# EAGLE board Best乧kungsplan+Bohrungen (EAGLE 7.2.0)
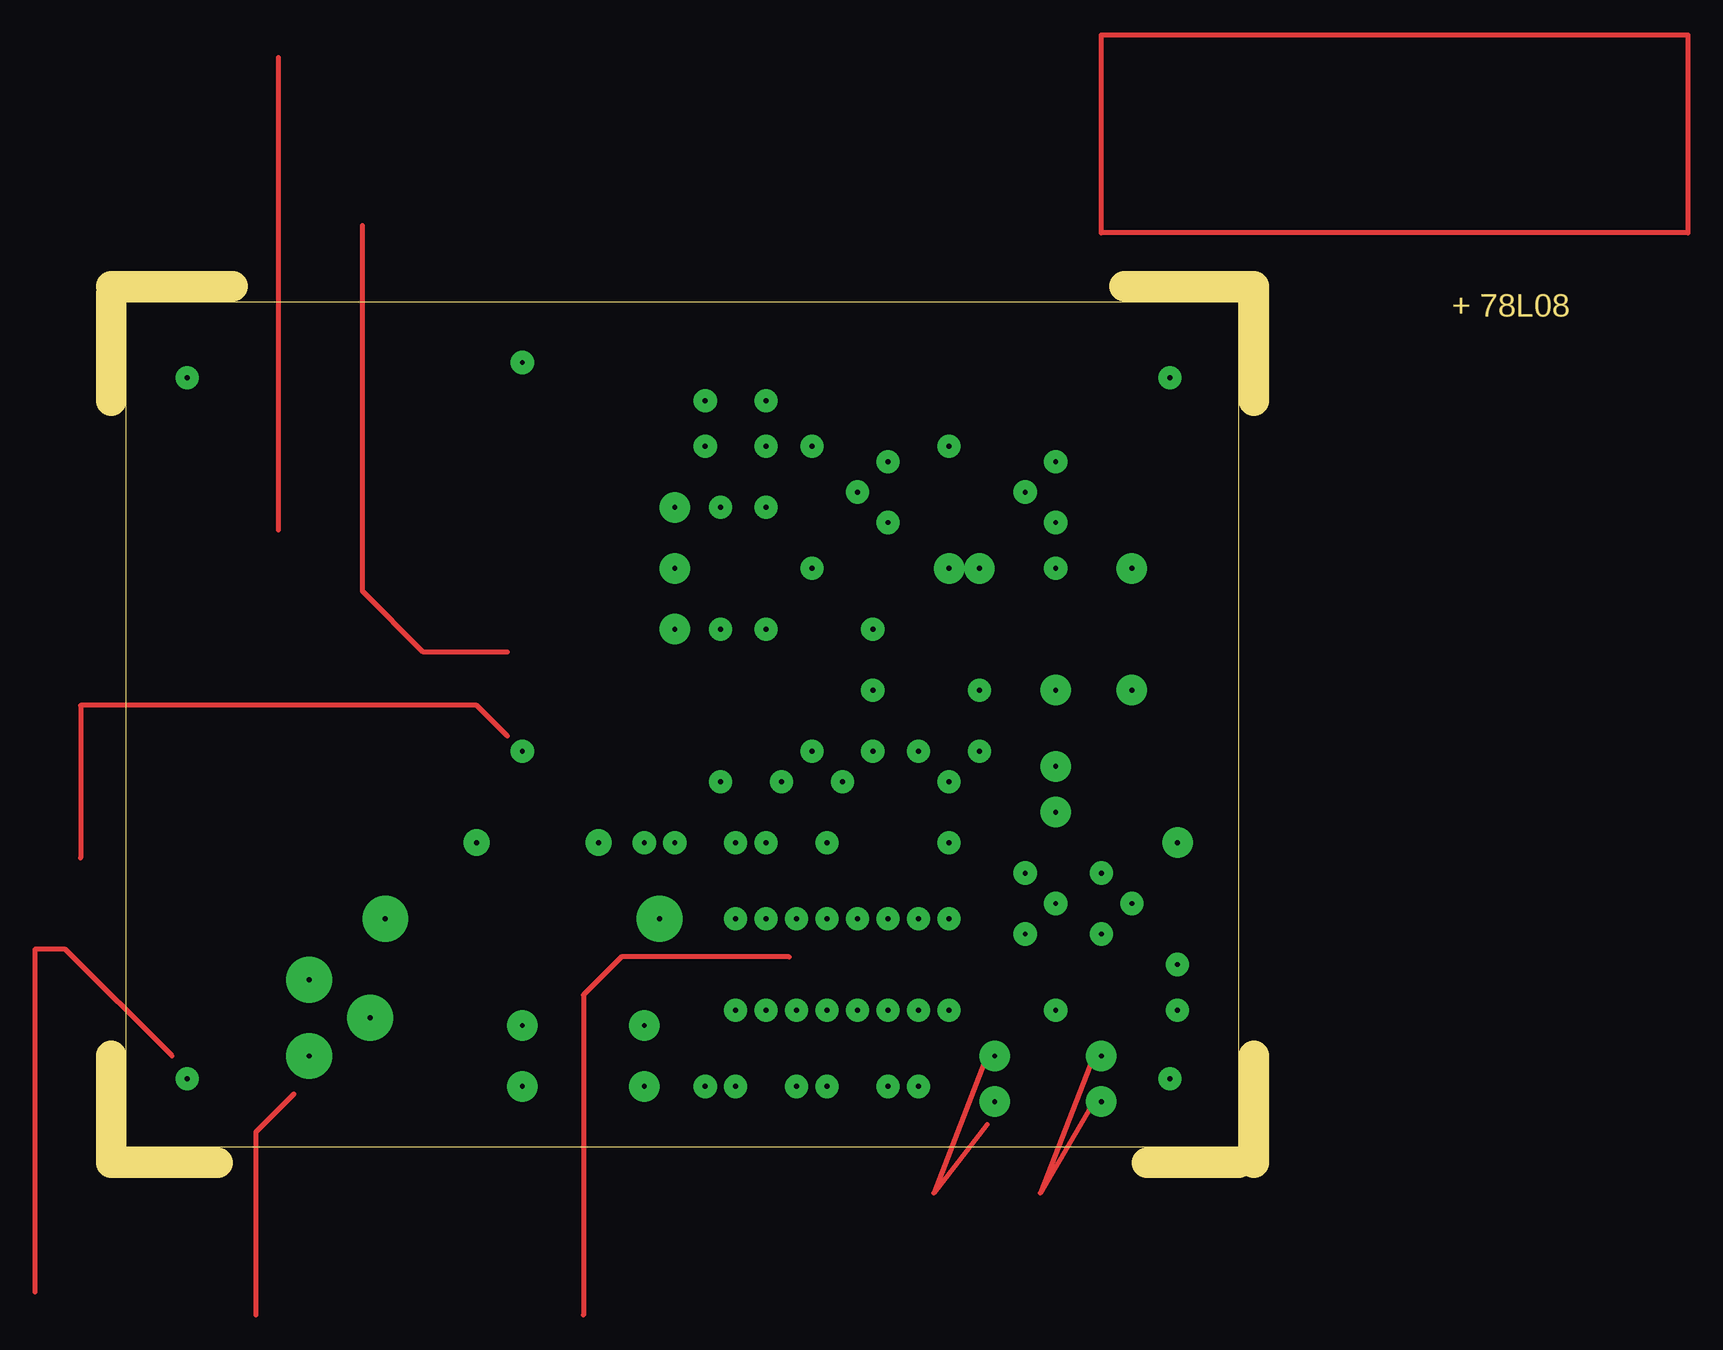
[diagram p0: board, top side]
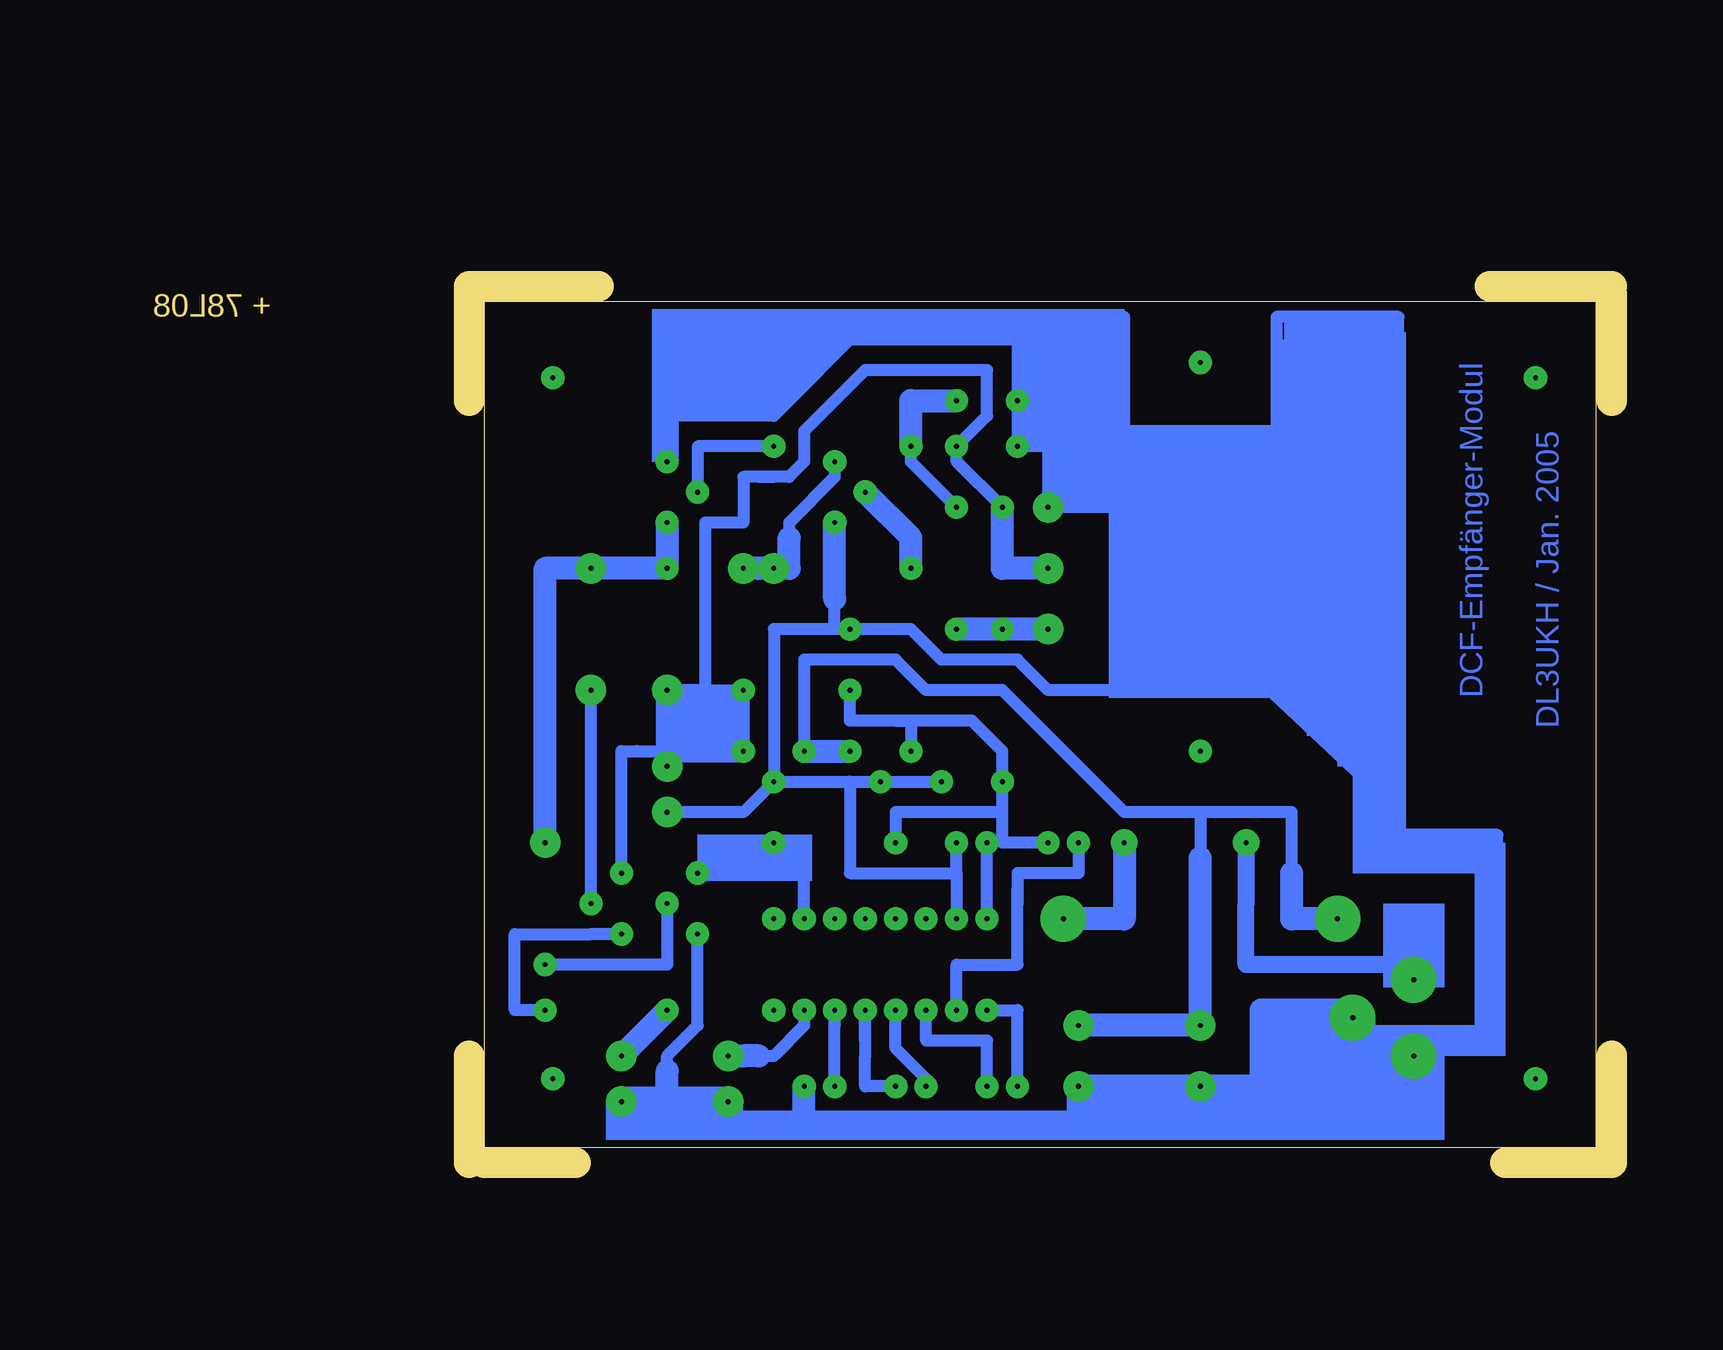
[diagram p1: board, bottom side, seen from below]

Size 95.25 x 73.02 mm. Coordinates in mm from the lower left corner, seen from the top.
Outline: 0,8.89 0,0 8.89,0
Outline: 0,72.39 0,63.5
Outline: 93.98,0 86.36,0
Outline: 95.25,0 95.25,8.89
Outline: 95.25,72.39 95.25,63.5
Outline: 0,73.02 10.16,73.02
Outline: 95.25,72.71 95.25,73.02 84.45,73.02
Outline: 1.27,71.75 93.98,71.75 93.98,1.27 1.27,1.27 1.27,71.75
Copper layers (1*16): Top 0.035mm / dielectric 1.5mm / Bottom 0.035mm
Design rules "default": minimum track width 10mil, minimum drill 24mil, track to track 8mil, track to pad 8mil, pad to pad 8mil, via to via 8mil, smd to smd 8mil, copper to edge 40mil, drill to drill 8mil, minimum pad ring 10mil, minimum via ring 8mil, stop-mask expansion 4mil, vias tented up to drill 0mil, thermal gap 10mil

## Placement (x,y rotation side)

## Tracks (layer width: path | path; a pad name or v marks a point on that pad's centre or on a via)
S$1  (via drill 0.41 pad 1.93)
  other vias: 6.35,6.98
S$2  (via drill 0.41 pad 1.93)
  other vias: 88.27,6.98
S$3  (via drill 0.41 pad 1.93)
  other vias: 88.27,65.41
S$4  (via drill 0.41 pad 1.93)
  other vias: 6.35,65.41
S$5
  Top 0.406: 33.02,42.55 26.04,42.55 20.95,47.62 20.95,78.1
S$6  (via drill 0.41 pad 2.18)
  Bottom 1.422: 16.51,16.51 30.48,16.51 30.48,21.59 v30.48,26.67
S$7  (via drill 0.41 pad 1.93)
  other vias: 34.29,34.29
S$8  (via drill 0.41 pad 1.93)
  other vias: 34.29,66.67
S$9  (via drill 0.41 pad 3.81)
  Bottom 1.93: v16.51,15.24 17.78,16.51
S$10
  Bottom 1.016: 11.43,10.79 14.61,10.79
S$11  (via drill 0.41 pad 3.81)
  other vias: 21.59,12.06
S$12  (via drill 0.41 pad 1.93)
  Bottom 1.016: v44.45,26.67 44.45,24.13 49.53,24.13 49.53,21.59 | 49.53,21.59 49.53,22.86 | v54.61,12.7 54.61,16.51 49.53,16.51 49.53,21.59
S$13  (via drill 0.41 pad 2.18, 0.41 pad 3.81)
  Bottom 1.93: v40.64,26.67 40.64,20.32 v45.72,20.32
S$14  (via drill 0.41 pad 1.93, 0.41 pad 2.54, 0.41 pad 3.81)
  Bottom 1.016: v63.5,34.29 v67.31,34.29 67.31,41.91 59.69,41.91 57.15,39.37 50.8,39.37 40.64,29.21 38.1,29.21 | 34.29,29.21 34.29,25.4 | 38.1,29.21 39.37,29.21 | 34.29,29.21 26.67,29.21 26.67,24.13 | 34.29,29.21 38.1,29.21
  Bottom 1.93: v44.45,11.43 v34.29,11.43 34.29,25.4 | v22.86,20.32 26.67,20.32 26.67,24.13 | v67.31,34.29 v63.5,34.29
S$15
  Bottom 1.93: 19.05,31.11 29.21,40.64
S$16  (via drill 0.41 pad 1.93, 0.41 pad 2.54)
  Bottom 1.016: v46.99,44.45 v50.8,44.45 v54.61,44.45
  Bottom 1.93: v46.99,44.45 v54.61,44.45
S$17  (via drill 0.41 pad 1.93)
  Bottom 1.93: v62.23,55.88 58.42,52.07 v58.42,49.53
S$18  (via drill 0.41 pad 1.93)
  Bottom 1.016: v52.07,6.35 52.07,10.16 57.15,10.16 v57.15,12.7
S$19  (via drill 0.41 pad 1.93)
  other vias: 76.2,19.05
S$20  (via drill 0.41 pad 1.93)
  Bottom 1.016: 64.77,11.43 v64.77,12.7 v64.77,6.35
S$21  (via drill 0.41 pad 1.93)
  Bottom 1.016: v54.61,54.61 58.42,58.42 v58.42,59.69
  Bottom 1.93: v54.61,63.5 58.42,63.5 v58.42,59.69
S$22  (via drill 0.41 pad 1.93, 0.41 pad 2.54, 0.41 pad 3.81)
  Bottom 1.016: 76.2,19.05 76.2,11.43 78.74,8.89 78.74,7.62 | 78.74,3.81 78.74,5.08 | 78.74,3.81 73.66,3.81 67.31,3.81 44.45,3.81 | 78.74,3.81 82.55,3.81 v82.55,5.08
  Bottom 1.93: 78.74,5.08 78.74,7.62 | 67.31,3.81 v67.31,6.35 | 44.45,5.08 v44.45,6.35 v34.29,6.35 | v82.55,5.08 v73.66,5.08 | 44.45,5.08 44.45,3.81 34.29,3.81 | 34.29,5.08 44.45,5.08 | 34.29,5.08 34.29,3.81 | 34.29,3.81 16.51,3.81 16.51,5.08 | 34.29,5.08 v34.29,6.35 | 16.51,6.35 29.21,6.35 | 29.21,6.35 v34.29,6.35 | 16.51,6.35 v16.51,8.89 | 16.51,5.08 21.59,5.08 | 21.59,5.08 34.29,5.08 | 16.51,5.08 16.51,6.35 | 21.59,5.08 21.59,7.62 | 21.59,12.06 21.59,12.7 29.21,12.7 29.21,6.35
  Bottom 2.54: 73.66,3.81 v73.66,5.08 v82.55,5.08 | 21.59,8.89 21.59,7.62
  Bottom 3.81: 21.59,12.06 21.59,8.89
S$23  (via drill 0.41 pad 1.93)
  other vias: 69.85,12.7
S$24  (via drill 0.41 pad 1.93)
  Bottom 1.016: v88.9,12.7 91.44,12.7 91.44,19.05 85.09,19.05 v82.55,19.05
S$25  (via drill 0.41 pad 1.93, 0.41 pad 2.54)
  Bottom 1.016: v85.09,21.59 v85.09,39.37
S$26  (via drill 0.41 pad 1.93)
  other vias: 57.15,20.32
S$27  (via drill 0.41 pad 1.93)
  other vias: 59.69,20.32
S$28  (via drill 0.41 pad 1.93)
  other vias: 62.23,20.32
S$29  (via drill 0.41 pad 1.93)
  other vias: 64.77,20.32
S$30  (via drill 0.41 pad 1.93)
  Bottom 1.016: v69.85,26.67 67.31,26.67 67.31,24.13 | v67.31,20.32 67.31,24.13 | 67.31,24.13 v76.2,24.13
S$31  (via drill 0.41 pad 1.93)
  other vias: 69.85,20.32
S$32  (via drill 0.41 pad 1.93)
  Bottom 1.016: v63.5,39.37 63.5,36.83 59.69,36.83 | v58.42,34.29 58.42,36.83 59.69,36.83 | 59.69,36.83 53.34,36.83 50.8,34.29 v50.8,31.75 50.8,29.21 | 50.8,29.21 50.8,26.67 v46.99,26.67 | 50.8,29.21 59.69,29.21 v59.69,26.67
S$33  (via drill 0.41 pad 1.93)
  Bottom 1.016: v52.07,20.32 v52.07,26.67
S$34
  Bottom 1.93: 66.67,69.21 71.12,64.77
S$35  (via drill 0.41 pad 1.93)
  Bottom 1.016: v59.69,12.7 59.69,9.53 57.15,6.98 v57.15,6.35
S$36  (via drill 0.41 pad 1.93)
  Bottom 1.016: v59.69,6.35 62.23,6.35 62.23,8.89 v62.23,12.7 62.23,10.16
S$37  (via drill 0.41 pad 1.93)
  Bottom 1.016: v49.53,6.35 49.53,12.7 v52.07,12.7
S$38  (via drill 0.41 pad 1.93)
  Bottom 1.016: v69.85,59.69 76.2,59.69 v76.2,55.88
S$39  (via drill 0.41 pad 1.93, 0.41 pad 2.54)
  Bottom 1.93: v88.9,26.67 88.9,49.53 v85.09,49.53 v78.74,49.53 v78.74,53.34
S$40  (via drill 0.41 pad 1.93, 0.41 pad 2.54)
  Bottom 1.016: v64.77,58.42 64.77,57.15 68.58,53.34 68.58,52.07 | 71.12,49.53 v72.39,49.53
  Bottom 1.93: v69.85,49.53 68.58,49.53 68.58,52.07 | v69.85,49.53 71.12,49.53 | v69.85,49.53 v72.39,49.53
S$41
  Bottom 1.93: 27.94,40.64 24.13,36.83
S$42  (via drill 0.41 pad 1.93)
  Bottom 1.016: v78.74,21.59 78.74,16.51 v88.9,16.51
S$43  (via drill 0.41 pad 1.93, 0.41 pad 2.54)
  Bottom 1.016: v67.31,12.7 67.31,11.43 69.85,8.89 71.12,8.89
  Bottom 1.93: 71.12,8.89 72.39,8.89 v73.66,8.89
S$44  (via drill 0.41 pad 1.93, 0.41 pad 2.54)
  Bottom 1.93: v78.74,12.7 v82.55,8.89
S$45  (via drill 0.41 pad 1.93, 0.41 pad 2.54)
  Bottom 1.016: 54.61,24.13 v54.61,26.67 | 54.61,24.13 v54.61,20.32 | 54.61,24.13 63.5,24.13 63.5,31.75 | v55.88,31.75 v60.96,31.75 63.5,31.75 | v78.74,29.21 72.39,29.21 v69.85,31.75 | v69.85,31.75 63.5,31.75 | v69.85,31.75 69.85,44.45 64.77,44.45 | 64.77,44.45 64.77,46.99 | 64.77,44.45 v63.5,44.45 58.42,44.45 55.88,41.91 49.53,41.91 46.99,39.37 40.64,39.37 40.64,40.64 | 78.74,63.5 73.66,68.58 69.85,68.58 | v49.53,63.5 v49.53,59.69 46.99,59.69 | 69.85,68.58 69.85,62.23 | 49.53,68.58 64.77,68.58 69.85,68.58 | 49.53,68.58 v49.53,63.5 | 46.99,63.5 v49.53,63.5 | 46.99,59.69 v46.99,54.61 40.64,54.61 | 46.99,59.69 46.99,63.5 | 40.64,54.61 39.37,54.61 | 40.64,54.61 46.99,59.69 | 46.99,68.58 46.99,63.5 | 46.99,68.58 49.53,68.58 | 46.99,68.58 40.64,68.58 40.64,60.96 | 40.64,60.96 40.64,57.15 40.64,70.48 78.74,70.48 | 40.64,60.96 27.94,60.96 27.94,70.48 17.78,70.48 17.78,27.3 9.53,27.3 9.53,12.7 | 69.85,62.23 62.23,69.85 | 69.85,62.23 78.74,62.23
  Bottom 1.93: 64.77,46.99 v64.77,53.34 | 78.74,63.5 78.74,62.23 v78.74,58.42 | 40.64,40.64 40.64,54.61 40.64,57.15 | 64.77,68.58 70.48,62.87
S$46
  Top 0.406: 56.52,17.14 42.55,17.14 39.37,13.97 39.37,-12.7
S$47  (via drill 0.41 pad 1.93, 0.41 pad 2.54)
  Bottom 1.016: 82.55,34.29 81.28,34.29 | v82.55,24.13 82.55,34.29 | v72.39,34.29 v72.39,39.37 75.56,39.37 | 75.56,39.37 v78.74,39.37 | 75.56,39.37 75.56,53.34 72.39,53.34 72.39,57.15 71.12,57.15 | 71.12,57.15 69.85,57.15 | 71.12,57.15 68.58,57.15 67.31,58.42 67.31,60.96 62.23,66.04 52.07,66.04 52.07,62.23 v54.61,59.69 54.61,58.42 v50.8,54.61 | 82.55,34.29 78.74,34.29
  Bottom 1.93: 78.74,34.29 v78.74,33.02 | v72.39,34.29 78.74,34.29 | v78.74,39.37 78.74,34.29 | v50.8,54.61 50.8,49.53 v46.99,49.53
S$48
  Bottom 1.016: 41.28,69.21 78.74,69.21
S$49
  Top 0.406: 73.02,8.89 68.58,-2.54 73.02,3.17
S$50
  Top 0.406: 81.91,8.89 77.47,-2.54 81.91,5.08
S$51
  Top 0.406: 33.02,35.56 30.48,38.1 -2.54,38.1 -2.54,25.4
S$52
  Top 0.406: 5.08,8.89 -3.81,17.78 -6.35,17.78 -6.35,-10.79
S$53
  Top 0.406: 13.97,52.71 13.97,92.08
S$54
  Top 0.406: 15.24,5.71 12.06,2.54 12.06,-12.7
S$55
  Top 0.406: 82.55,93.98 131.45,93.98 131.45,77.47 82.55,77.47 82.55,93.98
(copper drawn outside any net)
  shapes: Bottom area x42

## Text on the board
Bottom: DCF-Empfänger-Modul | DL3UKH / Jan. 2005
Pads: AUF BESTÜCKUNGS-SEITE GESEHEN
Dimension: + 78L08
tOrigins: Es ist keine Leiterplatten-Brücke notwendig ! | Freien Platz NICHT für Ferrit-Ant. | BOHRUNGEN | nutzen. Ant. außerhalb platzieren !!! | Alles mit 0,8mm bohren. | Anschluß-Drähte verlängern | alle Ausg. mit 1,0mm bohren | DCF-Empf.+MAX232 störten !! | Sicherung mit 1,4mm bohren | für Si-Halter | DCF-Ausg. + invert. DCF-Ausg. | an den Wechselschalter | 78L05 | 100n+zum Schalter | DCF- | Empfänger | C | 47n | BC547c | Masse | 47K | C | 110K | BC547c | +8 Volt | 33K | 110K | Ausg. | Eing. | DCF-Ausg. | 2K | 18K | 7,5K | 220µ | Masse | 2x | BC547+BC557 | 47n | Eing. | 78L05 | 78L08 | 220µ | 1N4002 | 1µ | 1µ | 2x Befestigung für DCF-Empf. | Bohrung 2,8mm für M2,7 Schrauben | mit Distanzhülse aus Plaste | 680 | C | C | BC557c | Sicherung 400mA | 30K | BC547c | MAX232 | 1 | 270 | C | E | 470µ | 47n | B | 1µ | 1µ | 1µ | 1N4002 | Printbuchse | 3x 2,0mm | RS232-Ausg. | LED gn 5mm | bohren und | alle Ausg. mit 1,0mm bohren | dann auffeilen | 4x Befestigungs- | Bohrungen 3,2mm und | Gehäuse-Nippel auch | auf 3,2mm aufbohren | für M3 Schraube | VORSICHT ! | IC mit Präzis.-Fassung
